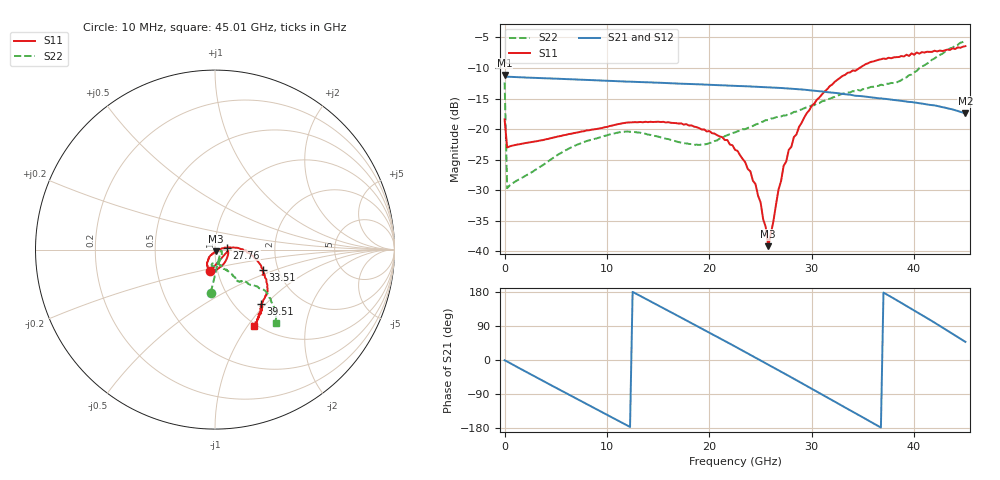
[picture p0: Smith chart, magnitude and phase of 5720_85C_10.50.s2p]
! Device:  ADRF5720
! Description: 0.5dB LSB GaAs MMIC 6-bit Digital Attenuator
! Frequency:  0.000009 -  40 GHz
! Ports:
!	RF1	= Port 1
!	RF2	= Port 2
! Vdd:  3.3 Volt
! Vss:  -3.3 Volt
! Control:  0/3.3 Volt
! State:  10.50 dB attenuation
! Data:  The device was measured using G-S-G Probes on a matrix board.
!  Data was collected using an calibrated 4 port network analyzer.
!  The reference plane for this measurement is at the launchers.
! Note:  Analog Devices supplies this data as a sample of measured data
!  for this product.  Your particular data for this product may vary.
!  Data was taken at 85 degrees C.
!  Analog Devices reserves the right to change this data at anytime.
# GHZ S DB R 45.0
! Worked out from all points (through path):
!   181 points, 10 MHz to 45.01 GHz, reference 45 ohm
!   highest |S21| = -11.12 dB at 10 MHz (marker M1); lowest = -17.4 dB at 45.01 GHz (marker M2)
!   group delay of S21, straight-line fit = 41 ps
!   lowest |S11| = -39.2 dB at 25.76 GHz (marker M3), VSWR 1.02, Z = 45.3 - j0.938 ohm
!   |S11| at or under -10 dB: start of sweep to 34.67 GHz
!   |S22| runs from -29.7 to -5.5 dB; largest |S21 - S12| = 0.0015
!   S11 on the Smith chart (normalised r, x): 10 MHz: 0.93, -0.22; 27.76 GHz: 1.14, +0.02; 33.51 GHz: 1.67, -0.40; 39.51 GHz: 1.30, -0.94; 45.01 GHz: 0.97, -1.07
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0.01  -18.41 -102.2  -11.12 -0.8  -11.11 -0.8  -12.36 -95.6
0.26  -23.02 -8.2  -11.42 -4.0  -11.42 -4.0  -29.67 -14.5
4.26  -21.61 -39.5  -11.70 -62.3  -11.69 -62.3  -25.28 -51.9
7.76  -20.35 -63.8  -11.93 -112.5  -11.92 -112.4  -22.11 -75.8
11.51  -19.05 -85.0  -12.19 -166.0  -12.18 -165.8  -20.44 -94.2
15.26  -18.84 -102.2  -12.42 140.4  -12.42 140.5  -21.36 -102.7
19.01  -19.84 -114.7  -12.67 86.5  -12.67 86.7  -22.60 -87.9
21.76  -21.79 -121.7  -12.86 46.7  -12.86 46.9  -20.99 -73.2
22.76  -23.57 -123.1  -12.94 32.1  -12.93 32.3  -20.35 -69.8
24.51  -28.99 -122.7  -13.06 6.5  -13.05 6.7  -19.26 -67.2
25.51  -36.00 -86.2  -13.13 -8.3  -13.12 -8.0  -18.53 -65.7
25.76  -39.16 -69.9  -13.15 -12.0  -13.15 -11.8  -18.53 -64.5
26.76  -29.90 2.8  -13.25 -27.0  -13.24 -26.7  -17.99 -62.3
27.26  -25.99 8.3  -13.30 -34.5  -13.29 -34.2  -17.77 -61.2
27.76  -23.39 9.2  -13.36 -42.0  -13.35 -41.7  -17.48 -60.3
28.76  -19.65 6.8  -13.49 -57.0  -13.48 -56.7  -16.92 -58.6
30.26  -15.80 -2.3  -13.72 -79.8  -13.71 -79.5  -16.08 -56.5
33.51  -10.78 -22.6  -14.33 -129.0  -14.32 -128.7  -14.03 -54.5
37.76  -8.40 -42.7  -15.18 166.2  -15.17 166.6  -12.44 -47.8
39.51  -8.02 -50.0  -15.55 138.9  -15.53 139.3  -11.16 -44.9
42.26  -7.29 -55.4  -16.21 94.1  -16.19 94.5  -8.08 -40.4
45.01  -6.42 -63.1  -17.43 47.9  -17.40 48.3  -5.49 -50.2
